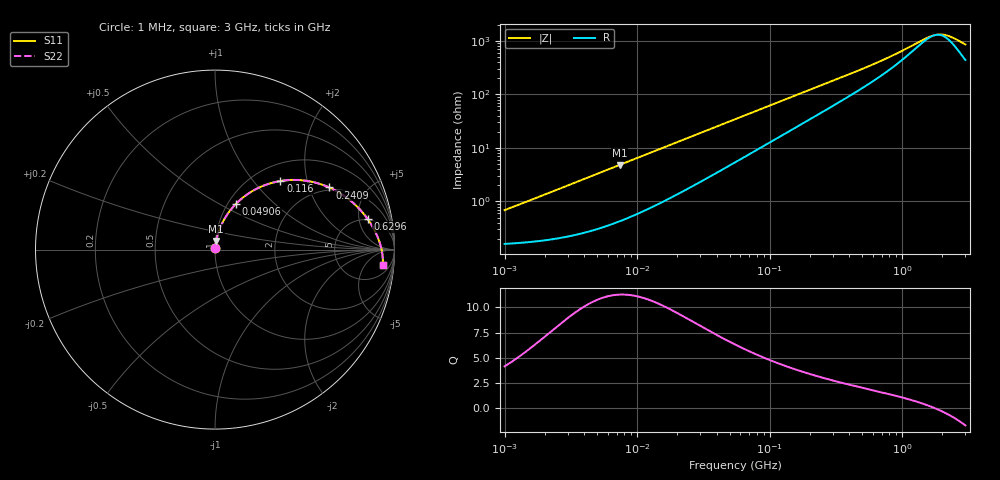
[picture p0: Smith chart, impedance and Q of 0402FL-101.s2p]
# MHz S MA R 50
!Freq  MagS11  AngS11  MagS21  AngS21  MagS12  AngS12  MagS22  AngS22
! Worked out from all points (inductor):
!   801 points, 1 MHz to 3 GHz, reference 50 ohm
!   read as one part in series: L = 106 nH near 1.041 MHz
!   highest Q = 11.3 at 7.401 MHz (marker M1), where L = 103 nH
!   self-resonance near 1.788 GHz
!   S11 on the Smith chart (normalised r, x): 1 MHz: 1.00, +0.01; 49.06 MHz: 1.09, +0.61; 116 MHz: 1.31, +1.39; 240.9 MHz: 1.89, +2.75; 629.6 MHz: 4.79, +6.61; 3 GHz: 10, -15
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1  0.006873 76.1  0.9984 -0.4  0.9984 -0.4  0.006873 76.1
3.823119  0.02514 82.8  0.9972 -1.4  0.9972 -1.4  0.02514 82.8
7.400828  0.04795 82.2  0.9946 -2.7  0.9946 -2.7  0.04795 82.2
14.47069  0.09192 79.2  0.987 -5.2  0.987 -5.2  0.09192 79.2
28.86629  0.1766 73.0  0.9633 -10.1  0.9633 -10.1  0.1766 73.0
49.06256  0.2827 65.2  0.918 -16.2  0.918 -16.2  0.2827 65.2
54.77226  0.3098 63.2  0.9036 -17.8  0.9036 -17.8  0.3098 63.2
78.52918  0.4094 55.7  0.8405 -23.7  0.8405 -23.7  0.4094 55.7
116.0221  0.5279 46.4  0.7417 -31.0  0.7417 -31.0  0.5279 46.4
155.0909  0.6138 39.1  0.6509 -36.5  0.6509 -36.5  0.6138 39.1
209.4008  0.6929 31.7  0.5491 -41.6  0.5491 -41.6  0.6929 31.7
240.8952  0.7251 28.5  0.5014 -43.6  0.5014 -43.6  0.7251 28.5
381.7355  0.8086 19.2  0.3556 -48.4  0.3556 -48.4  0.8086 19.2
629.6259  0.867 11.4  0.2276 -48.8  0.2276 -48.8  0.867 11.4
792.5923  0.8859 8.5  0.1799 -46.5  0.1799 -46.5  0.8859 8.5
1519.029  0.922 1.6  0.08243 -18.2  0.08243 -18.2  0.922 1.6
1678.92  0.9259 0.6  0.07486 -7.7  0.07486 -7.7  0.9259 0.6
1818.868  0.9286 -0.2  0.07144 2.2  0.07144 2.2  0.9286 -0.2
2010.32  0.9317 -1.2  0.07107 15.4  0.07107 15.4  0.9317 -1.2
2221.924  0.9343 -2.2  0.07523 28.1  0.07523 28.1  0.9343 -2.2
2455.801  0.9365 -3.2  0.08353 38.9  0.08353 38.9  0.9365 -3.2
3000  0.9393 -5.4  0.1098 53.8  0.1098 53.8  0.9393 -5.4
